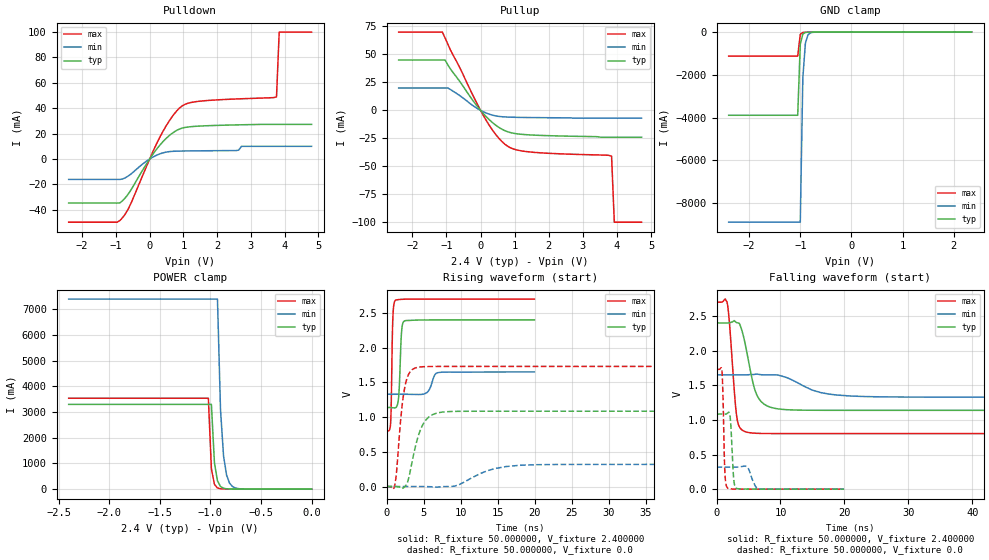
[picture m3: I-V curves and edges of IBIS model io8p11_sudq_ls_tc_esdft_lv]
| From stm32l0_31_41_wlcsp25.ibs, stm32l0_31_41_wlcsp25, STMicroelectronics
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|   Model io8p11_sudq_ls_tc_esdft_lv
[Model]  io8p11_sudq_ls_tc_esdft_lv
Model_type I/O
Polarity   Non-Inverting
Enable   Active-Low
Vinl =   0.720000V
Vinh =   1.680000V
Vmeas =  1.200000V
Cref =   50.000000pF
Rref =   100.000000M
Vref =   0.0V
C_comp   2.242700pF   2.201100pF   2.304400pF
[Temperature Range]   25.000000   0.125000k   -40.000000
[Pullup Reference]   2.400000V   1.650000V   2.700000V
[Pulldown Reference]   0.0V   0.0V   0.0V
[POWER Clamp Reference]   2.400000V   1.650000V   2.700000V
[GND Clamp Reference]   0.0V   0.0V   0.0V
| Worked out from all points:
|   slope of the pulldown table from 0 to 0.36 V, typ, clamps not added: 28.4 ohm
|   slope of the pullup table from 0 to 0.36 V, typ, clamps not added: 32.2 ohm
|   GND clamp passes 1 mA (typ) near -0.65 V on its own axis
|   POWER clamp passes 1 mA (typ) near -0.63 V on its own axis
|   rising waveform, R_fixture 50.000000, V_fixture 2.400000: 20-80 % time 281ps typ, 655ps min, 189ps max; typ from 1.14 V to 2.4 V
|   rising waveform, R_fixture 50.000000, V_fixture 0.0: 20-80 % time 1.6ns typ, 4.04ns min, 929ps max; typ from 0 V to 1.08 V
|   falling waveform, R_fixture 50.000000, V_fixture 2.400000: 20-80 % time 1.8ns typ, 4.77ns min, 909ps max; typ from 2.4 V to 1.14 V
|   falling waveform, R_fixture 50.000000, V_fixture 0.0: 20-80 % time 358ps typ, 795ps min, 265ps max; typ from 1.08 V to 0 V
[Pulldown]
|Voltage   I(typ)   I(min)   I(max)
-2.4V     -34.7mA    -16.08mA   -49.77mA
-880mV    -34.55mA   -16.08mA   -48.41mA
-560mV    -24.66mA   -11.95mA   -35.31mA
240mV     8.893mA    3.395mA    13.9mA
560mV     17.98mA    5.759mA    29.16mA
880mV     23.57mA    6.247mA    40.03mA
1.44V     25.89mA    6.452mA    45.41mA
2.56V     26.87mA    6.65mA     47.29mA
2.72V     26.96mA    10mA       47.46mA
3.76V     27.3mA     10mA       49mA
3.84V     27.3mA     10mA       100mA
4.8V      27.3mA     10mA       100mA
[Pullup]
|Voltage   I(typ)   I(min)   I(max)
-2.4V     45mA       20mA       70mA
-1.12V    45mA       20mA       70mA
-1.04V    45mA       20mA       64.8mA
-880mV    36.92mA    18.6mA     53.87mA
80mV      -2.838mA   -1.235mA   -4.478mA
480mV     -14.04mA   -5.139mA   -22.91mA
800mV     -19.2mA    -6.004mA   -32.18mA
1.04V     -20.85mA   -6.221mA   -35.23mA
1.44V     -21.93mA   -6.415mA   -37.19mA
3.84V     -24mA      -7mA       -41mA
3.92V     -24mA      -7mA       -100mA
4.72V     -24mA      -7mA       -100mA
[GND_clamp]
|Voltage   I(typ)   I(min)   I(max)
-2.4V     -3.892A    -8.896A    -1.127A
-1.05V    -3.892A    -8.896A    -1.127A
-1V       -568.8mA   -8.896A    -105.4mA
-950mV    -88.95mA   -2.143A    -18.03mA
-900mV    -18.15mA   -522.9mA   -8.959mA
-850mV    -6.699mA   -130.7mA   -6.568mA
-800mV    -4.014mA   -34.5mA    -4.858mA
-600mV    -514.6uA   -842.9uA   -496.4uA
2.35V     0A         0A         0A
[POWER_clamp]
|Voltage   I(typ)   I(min)   I(max)
-2.4V     3.303A     7.406A     3.542A
-1.02V    3.303A     7.406A     3.542A
-990mV    3.303A     7.406A     802.4mA
-960mV    1.032A     7.406A     186.5mA
-930mV    325.2mA    7.406A     47.59mA
-900mV    104.8mA    3.098A     15.78mA
-870mV    35.83mA    1.298A     8.015mA
-840mV    13.93mA    544.8mA    5.668mA
-810mV    6.712mA    229.8mA    4.56mA
-750mV    2.922mA    42.35mA    3.077mA
-690mV    1.741mA    8.856mA    1.91mA
0V        0A         0A         0A
[Ramp]
| variable   typ   min   max
dV/dt_r  0.65070/1.59665n   0.19118/4.03813n   1.03800/0.92607n
dV/dt_f  0.75696/1.80064n   0.19272/4.76133n   1.13786/0.90681n
R_load = 50.000000
[Rising Waveform]
R_fixture= 50.000000
V_fixture= 2.400000
V_fixture_min= 1.650000
V_fixture_max= 2.700000
|time   V(typ)   V(min)   V(max)
0s        1.139V     1.329V     802.4mV
560.6ps   1.138V     1.329V     929.3mV
840.8ps   1.135V     1.329V     2.393V
1.201ns   1.134V     1.329V     2.682V
1.602ns   1.255V     1.329V     2.692V
2.042ns   2.248V     1.329V     2.696V
2.402ns   2.383V     1.329V     2.698V
5.285ns   2.399V     1.343V     2.7V
7.047ns   2.4V       1.642V     2.7V
19.94ns   2.4V       1.65V      2.7V
[Rising Waveform]
R_fixture= 50.000000
V_fixture= 0.0
V_fixture_min= 0.0
V_fixture_max= 0.0
|time   V(typ)   V(min)   V(max)
0s        1.007uV    6.375uV    233.6uV
1.126ns   -47.89uV   1.883uV    29.52mV
2.002ns   -17.57mV   -4.394uV   1.066V
2.377ns   -9.6mV     12.57uV    1.38V
3.003ns   125.8mV    76.7uV     1.622V
4.004ns   621.3mV    76.62uV    1.711V
5.506ns   981.8mV    -1.804mV   1.728V
8.383ns   1.079V     56.39uV    1.73V
18.14ns   1.085V     306.6mV    1.73V
62.31ns   1.085V     318.6mV    1.73V
[Falling Waveform]
R_fixture= 50.000000
V_fixture= 2.400000
V_fixture_min= 1.650000
V_fixture_max= 2.700000
|time   V(typ)   V(min)   V(max)
0s        2.4V       1.65V      2.7V
1.627ns   2.4V       1.65V      2.707V
2.002ns   2.401V     1.65V      2.42V
3.128ns   2.406V     1.65V      1.071V
3.504ns   2.4V       1.65V      912.6mV
4.505ns   2.086V     1.65V      830mV
6.381ns   1.346V     1.661V     806.3mV
9.259ns   1.165V     1.65V      802.8mV
20.77ns   1.139V     1.346V     802.4mV
62.31ns   1.139V     1.329V     802.4mV
[Falling Waveform]
R_fixture= 50.000000
V_fixture= 0.0
V_fixture_min= 0.0
V_fixture_max= 0.0
|time   V(typ)   V(min)   V(max)
0s        1.085V     318.6mV    1.73V
840.8ps   1.085V     318.6mV    1.712V
1.001ns   1.084V     318.6mV    1.366V
1.281ns   1.084V     318.6mV    292.1mV
1.722ns   1.098V     318.6mV    17.63mV
2.122ns   1.047V     318.6mV    3.891mV
2.683ns   152.9mV    318.3mV    2.132mV
3.123ns   12mV       318.4mV    1.574mV
6.607ns   635.3uV    5.943mV    296.4uV
19.94ns   1.007uV    6.375uV    233.6uV
